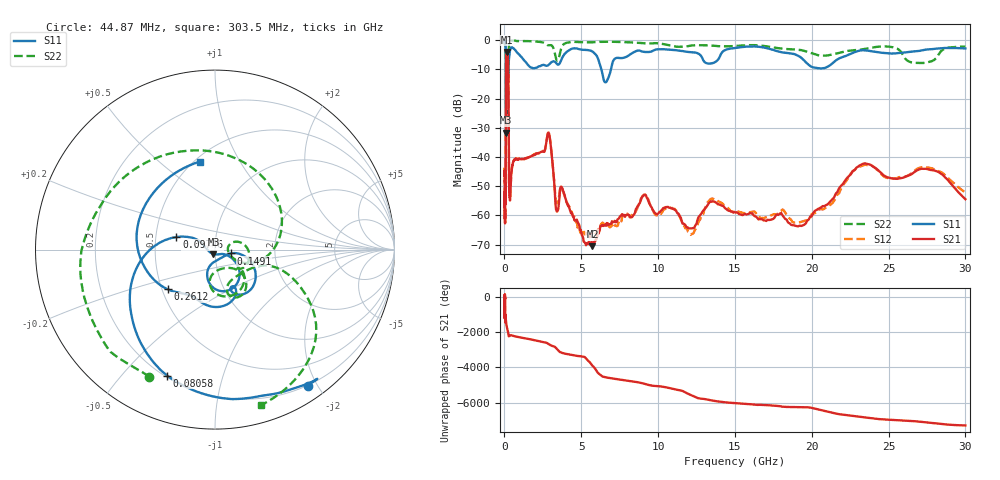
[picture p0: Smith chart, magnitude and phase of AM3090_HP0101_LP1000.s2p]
! Date/Time: Thu, Feb 28, 2019 1:58 PM
! Network Analyzer: Agilent Technologies E8364B Rev: A.07.50.67
! Sweep from 0.010 to 30.000 GHz, 1601 Points, Sweep Type: LOG
! Power Supply: 5.023 V, 0.002 A
# Hz S DB R 50
!freq MagS11 AngS11 MagS21 AngS21 MagS12 AngS12 MagS22 AngS22
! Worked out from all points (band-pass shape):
!   1601 points, 10 MHz to 30 GHz, reference 50 ohm
!   highest |S21| = -4.03 dB at 154.4 MHz (marker M1); lowest = -70.5 dB at 5.725 GHz (marker M2)
!   |S21| within 3 dB of the highest: 107.6 MHz to 239.5 MHz (131.9 MHz wide, 76 % of centre)
!   lowest |S11| = -31.7 dB at 105.1 MHz (marker M3), VSWR 1.05, Z = 49.1 - j2.41 ohm
!   |S11| at or under -10 dB: 95.9 MHz to 225 MHz (129.1 MHz wide, 80.4 % of centre); 232.4 MHz to 256.6 MHz (24.17 MHz wide, 9.89 % of centre); 6.308 GHz to 6.931 GHz (623.3 MHz wide, 9.42 % of centre)
!   |S22| runs from -22.9 to -0.1 dB; largest |S21 - S12| = 0.0095
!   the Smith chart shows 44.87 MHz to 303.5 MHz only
!   S11 on the Smith chart (normalised r, x): 44.87 MHz: 0.20, -1.87; 80.58 MHz: 0.21, -0.67; 97.46 MHz: 0.64, +0.10; 149.1 MHz: 1.19, -0.05; 261.2 MHz: 0.53, -0.27; 303.5 MHz: 0.53, +0.69
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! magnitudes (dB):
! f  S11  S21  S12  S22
! 10 MHz  -0.2  -46.4  -44.9  -0.6
! 38.04 MHz  -0.5  -62.2  -57.7  -1.5
! 44.87 MHz  -0.7  -55.3  -58.5  -2.0
! 80.58 MHz  -2.5  -48.8  -48.9  -4.8
! 97.46 MHz  -12.9  -15.4  -15.3  -11.5
! 105.1 MHz  -31.7  -8.0  -8.0  -22.2
! 120.9 MHz  -12.6  -5.2  -5.2  -15.4
! 144.7 MHz  -24.6  -4.1  -4.1  -15.8
! 149.1 MHz  -20.9  -4.1  -4.0  -15.5
! 154.4 MHz  -15.5  -4.0  -4.0  -14.5
! 261.2 MHz  -9.3  -15.2  -15.2  -9.8
! 303.5 MHz  -6.1  -50.7  -49.6  -0.9
! 550.5 MHz  -2.7  -42.0  -41.8  -0.2
! 2.084 GHz  -9.5  -38.8  -38.8  -0.5
! 2.884 GHz  -8.4  -31.8  -31.7  -1.8
! 3.402 GHz  -8.1  -58.6  -55.6  -6.9
! 5.725 GHz  -3.9  -70.5  -66.0  -0.8
! 6.619 GHz  -14.4  -63.5  -62.8  -0.6
! 7.926 GHz  -5.8  -59.9  -59.1  -0.7
! 19.22 GHz  -5.7  -63.5  -62.3  -3.4
! 23.48 GHz  -3.5  -42.2  -42.6  -3.0
! 30 GHz  -2.9  -54.4  -52.1  -2.2
